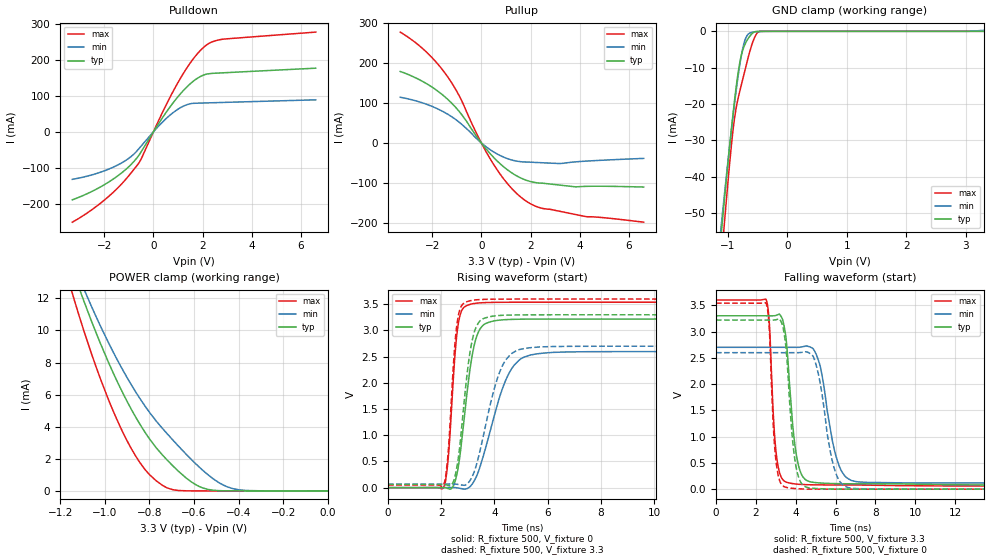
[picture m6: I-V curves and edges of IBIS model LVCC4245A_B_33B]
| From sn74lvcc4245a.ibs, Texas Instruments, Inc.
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[Model]   LVCC4245A_B_33B
Model_type  I/O
Vinl=0.8
Vinh=2.0
Enable   Active-Low
Vref =   0
Rref =   500
Cref =   50p
Vmeas =   1.5
| variable   typ   min   max
C_comp   11.0pF   NA   NA
| C_pullup   10.10pF   6.76pF   11.57pF
| C_pulldown   8.38pF   6.99pF   10.02pF
| C_tri-state   6.08pF   5.36pF   7.16pF
[Temperature Range]   40   100   -40
| Ambient temperature   25   85   -40
[Voltage range]   3.3   2.7   3.6
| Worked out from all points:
|   slope of the pulldown table from 0 to 0.495 V, typ, clamps not added: 9.51 ohm
|   slope of the pullup table from 0 to 0.495 V, typ, clamps not added: 13.8 ohm
|   GND clamp passes 1 mA (typ) near -0.61 V on its own axis
|   POWER clamp passes 1 mA (typ) near -0.65 V on its own axis
|   rising waveform, R_fixture 500, V_fixture 0: 20-80 % time 472ps typ, 917ps min, 281ps max; typ from 0 V to 3.22 V
|   falling waveform, R_fixture 500, V_fixture 3.3: 20-80 % time 439ps typ, 721ps min, 286ps max; typ from 3.3 V to 0.062 V
|   rising waveform, R_fixture 500, V_fixture 3.3: 20-80 % time 427ps typ, 768ps min, 267ps max; typ from 0.059 V to 3.3 V
|   falling waveform, R_fixture 500, V_fixture 0: 20-80 % time 389ps typ, 651ps min, 263ps max; typ from 3.22 V to 0 V
[GND Clamp]
| LVCC4245A_B_33B
|   Voltage   I(typ)   I(min)   I(max)
-3.3V     -499.6mA   -462mA     -562mA
-1.115V   -56.35mA   -54.02mA   -64.13mA
-1.09V    -51.92mA   -49.98mA   -59.1mA
-1.07V    -48.4mA    -46.79mA   -55.13mA
-1.05V    -44.93mA   -43.64mA   -51.21mA
-915mV    -22.93mA   -23.52mA   -27.44mA
-825mV    -11.08mA   -11.99mA   -18.22mA
-725mV    -4.044mA   -3.056mA   -11.52mA
-635mV    -1.412mA   -504.5uA   -5.741mA
-550mV    -124.6uA   -154.6uA   -1.652mA
-465mV    -7.252uA   -63.87uA   -16.58uA
3.3V      24.21pA    285.9uA    451.3pA
[POWER Clamp]
| LVCC4245A_B_33B
|   Voltage   I(typ)   I(min)   I(max)
-3.3V     175.8mA    151.7mA    218.9mA
-1.155V   14.22mA    14.67mA    12.76mA
-1.135V   13.42mA    13.97mA    11.82mA
-1.095V   11.88mA    12.63mA    10.03mA
-1.06V    10.59mA    11.51mA    8.564mA
-985mV    8.06mA     9.28mA     5.741mA
-915mV    5.983mA    7.426mA    3.537mA
-820mV    3.659mA    5.292mA    1.338mA
-740mV    2.215mA    3.872mA    332.8uA
-595mV    409.7uA    1.726mA    1.993uA
-450mV    4.406uA    248.1uA    115.3nA
-48.03fV  24.98pA    222.8pA    557.7pA
[Pulldown]
| LVCC4245A_B_33B
|   Voltage   I(typ)   I(min)   I(max)
-3.3V     -189.5mA   -132.4mA   -251.8mA
-1.805V   -139.3mA   -103.5mA   -179mA
-1.115V   -104.2mA   -79.13mA   -131.5mA
-650mV    -70.66mA   -51.58mA   -92.12mA
-480mV    -53.4mA    -38.07mA   -72.87mA
285mV     30.75mA    21.32mA    42.31mA
920mV     91.25mA    59.39mA    127.8mA
1.56V     137.5mA    78.78mA    197.8mA
2.12V     159.8mA    80.34mA    239.8mA
2.395V    162.7mA    80.89mA    250.8mA
2.84V     164.3mA    81.78mA    258.1mA
6.6V      177.2mA    89mA       277.7mA
[Pullup]
| LVCC4245A_B_33B
|   Voltage   I(typ)   I(min)   I(max)
-3.3V     179.4mA    114.8mA    278.2mA
-2.305V   151.5mA    98.73mA    232.2mA
-1.47V    115mA      75.75mA    174.5mA
-910mV    79.62mA    52.51mA    119.3mA
-145mV    12.06mA    7.966mA    17.6mA
440mV     -32.36mA   -20.18mA   -48.09mA
1.055V    -67.13mA   -39.15mA   -101.6mA
1.665V    -89.58mA   -47.33mA   -138.9mA
2.09V     -98.13mA   -48.5mA    -155.5mA
2.515V    -101.1mA   -49.72mA   -164.5mA
3.825V    -110mA     -47.42mA   -179.4mA
6.6V      -110.5mA   -38.67mA   -198.7mA
[Ramp]
| LVCC4245A_B_33B
| variable   typ   min   max
dV/dt_r   1.95/4.82E-10   1.58/9.30E-10   2.14/2.87E-10
dV/dt_f   1.96/4.60E-10   1.58/7.59E-10   2.14/2.98E-10
R_load = 500
[Rising Waveform]
| LVCC4245A_B_33B
R_fixture =   500
C_fixture =   0
L_fixture =   0
V_fixture =   0
V_fixture_min = 0
V_fixture_max = 0
|   Time   V(typ)   V(min)   V(max)
0s        145.5pV    4.16nV     446.8pV
2.095ns   2.072mV    34.98uV    5.23mV
2.26ns    -18.76mV   1.321mV    544.6mV
2.51ns    102.6mV    1.378mV    2.491V
2.65ns    426.5mV    -7.971mV   3.152V
3.265ns   2.77V      152.5mV    3.518V
3.61ns    3.115V     654mV      3.532V
4.56ns    3.21V      2.195V     3.539V
5.82ns    3.218V     2.568V     3.54V
50ns      3.219V     2.598V     3.54V
[Falling Waveform]
| LVCC4245A_B_33B
R_fixture =   500
C_fixture =   0
L_fixture =   0
V_fixture =   3.3
V_fixture_min = 2.7
V_fixture_max = 3.6
|   Time   V(typ)   V(min)   V(max)
0s        3.3V       2.7V       3.6V
2.52ns    3.3V       2.7V       3.602V
3.055ns   3.313V     2.7V       576.2mV
3.46ns    3.013V     2.7V       146.2mV
3.735ns   1.771V     2.7V       113.1mV
4.365ns   230.1mV    2.712V     88.05mV
5.185ns   118.9mV    2.396V     81.38mV
6.195ns   104.4mV    426.4mV    79.82mV
7.1ns     101.7mV    139.3mV    78.87mV
50ns      62.21mV    86.34mV    47.99mV
[Rising Waveform]
| LVCC4245A_B_33B
R_fixture =   500
C_fixture =   0
L_fixture =   0
V_fixture =   3.3
V_fixture_min = 2.7
V_fixture_max = 3.6
|   Time   V(typ)   V(min)   V(max)
0s        58.59mV    67.64mV    46.85mV
2.095ns   60.55mV    67.69mV    59.91mV
2.25ns    42.82mV    68.81mV    610.7mV
2.485ns   156.4mV    69.27mV    2.55V
2.61ns    458.6mV    62.96mV    3.189V
3.005ns   2.307V     86.88mV    3.557V
3.205ns   2.899V     257mV      3.579V
4.265ns   3.289V     2.289V     3.599V
5.35ns    3.299V     2.671V     3.6V
50ns      3.3V       2.7V       3.6V
[Falling Waveform]
| LVCC4245A_B_33B
R_fixture =   500
C_fixture =   0
L_fixture =   0
V_fixture =   0
V_fixture_min = 0
V_fixture_max = 0
|   Time   V(typ)   V(min)   V(max)
0s        3.219V     2.598V     3.54V
2.515ns   3.219V     2.598V     3.536V
3.01ns    3.225V     2.598V     533.8mV
3.585ns   2.334V     2.597V     29.02mV
3.885ns   773.6mV    2.598V     14.18mV
4.235ns   141.2mV    2.6V       5.378mV
4.925ns   15.22mV    2.482V     917.2uV
5.91ns    2.172mV    422.9mV    234.4uV
6.73ns    532uV      22.15mV    191.5uV
50ns      50.53uV    17.45uV    14.12uV
